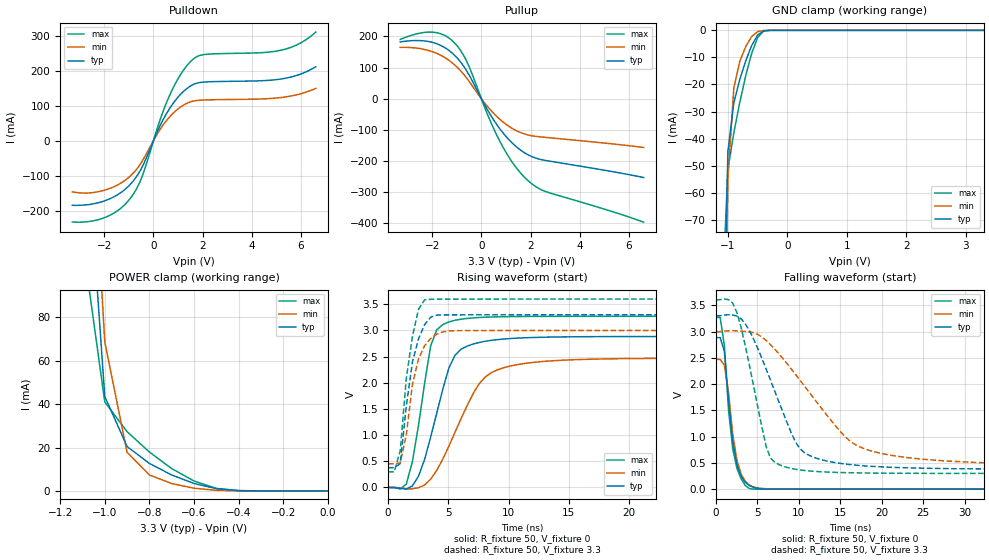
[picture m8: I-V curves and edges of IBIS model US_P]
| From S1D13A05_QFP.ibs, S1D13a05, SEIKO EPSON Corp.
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[Model]   US_P
Model_type I/O
Enable Active-Low
Polarity Non-Inverting
Vinh=2.0
Vinl=0.8
Vref=0
Vmeas=1.65
Rref=500
Cref=100pf
C_comp   5p   4p   6p
[Temperature Range] 25   85   -40
[Voltage Range]   3.3   3.0   3.6
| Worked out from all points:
|   slope of the pulldown table from 0 to 0.495 V, typ, clamps not added: 6.74 ohm
|   slope of the pullup table from 0 to 0.495 V, typ, clamps not added: 7.33 ohm
|   GND clamp passes 1 mA (typ) near -0.45 V on its own axis
|   POWER clamp passes 1 mA (typ) near -0.50 V on its own axis
|   falling waveform, R_fixture 50, V_fixture 0: 20-80 % time 1.22ns typ, 1.25ns min, 1.12ns max; typ from 2.88 V to 0 V
|   falling waveform, R_fixture 50, V_fixture 3.3: 20-80 % time 4.47ns typ, 7.76ns min, 2.62ns max; typ from 3.3 V to 0.379 V
|   rising waveform, R_fixture 50, V_fixture 0: 20-80 % time 2.02ns typ, 3.12ns min, 1.33ns max; typ from 0 V to 2.88 V
|   rising waveform, R_fixture 50, V_fixture 3.3: 20-80 % time 1.14ns typ, 1.12ns min, 971ps max; typ from 0.378 V to 3.3 V
[Pullup]
-3.3V     182mA      164.8mA    189.8mA
-2.6V     186.7mA    161.9mA    208.6mA
-2V       180.8mA    151.1mA    213.4mA
-1.5V     164.5mA    132.5mA    203.4mA
-1.1V     140.1mA    109.3mA    179.6mA
-600mV    89.77mA    66.62mA    120.5mA
300mV     -42.81mA   -29.74mA   -59.99mA
900mV     -111.5mA   -75.9mA    -158.2mA
1.5V      -159.1mA   -105.3mA   -229.4mA
2.1V      -187.1mA   -119.5mA   -275.7mA
2.7V      -199.1mA   -124.6mA   -300mA
6.6V      -252.7mA   -156.2mA   -395.8mA
[Pulldown]
-3.3V     -184.8mA   -146.4mA   -232.6mA
-1.9V     -169.9mA   -139.8mA   -217.7mA
-900mV    -121.6mA   -98.26mA   -161.1mA
-500mV    -80.82mA   -63.36mA   -109.6mA
300mV     47.55mA    35.72mA    66.22mA
700mV     96.96mA    71.67mA    136.6mA
1.1V      132.7mA    96.38mA    189.3mA
1.6V      160.5mA    113.3mA    232.8mA
2.1V      168.2mA    116.8mA    247mA
5.2V      176.9mA    123.8mA    259.4mA
5.9V      188.8mA    132.9mA    276.9mA
6.6V      211.7mA    149.8mA    311.1mA
[GND Clamp]
-3.3V     -5.912A    -5.005A    -7.437A
-1.1V     -148.8mA   -201.2mA   -101.3mA
-1V       -44.75mA   -55.01mA   -51.59mA
-900mV    -26.74mA   -21.22mA   -37.75mA
-800mV    -18.11mA   -11.47mA   -26.61mA
-700mV    -11.25mA   -5.992mA   -16.74mA
-600mV    -5.634mA   -2.285mA   -8.486mA
-500mV    -1.764mA   -477.5uA   -2.648mA
-400mV    -228.7uA   -55.77uA   -273.5uA
-300mV    -14.09uA   -4.898uA   -8.486uA
3.3V      997.8pA    2.959uA    138.9pA
[POWER Clamp]
-3.3V     6.221A     5.265A     7.806A
-1.1V     190.4mA    247mA      115.3mA
-1V       43.51mA    68.6mA     40.98mA
-900mV    20.45mA    17.8mA     27.29mA
-800mV    12.66mA    7.365mA    17.91mA
-700mV    7.343mA    3.399mA    10.28mA
-600mV    3.431mA    1.245mA    4.569mA
-500mV    1.039mA    278.7uA    1.157mA
-400mV    155.6uA    36.37uA    108uA
0V        997.8pA    2.129nA    167.6pA
[Falling Waveform]
R_fixture=50
V_fixture=0
V_fixture_min=0
V_fixture_max=0
0s        2.885V     2.471V     3.271V
505.1ps   2.885V     2.471V     3.27V
1.01ns    2.63V      2.363V     2.739V
1.515ns   1.701V     1.838V     1.505V
2.02ns    902.7mV    1.05V      770.1mV
2.525ns   472.3mV    551.8mV    397.7mV
3.03ns    247.6mV    286.4mV    199.1mV
4.04ns    66.95mV    79.7mV     10.84mV
7.576ns   1.173mV    2.989mV    758.1uV
50ns      4.747uV    28.51uV    6.901uV
[Falling Waveform]
R_fixture=50
V_fixture=3.3
V_fixture_min=3.0
V_fixture_max=3.6
0s        3.3V       3V         3.6V
1.515ns   3.321V     3.015V     3.609V
2.525ns   3.294V     3.014V     3.362V
4.04ns    3.016V     2.995V     2.354V
6.061ns   2.286V     2.831V     810.9mV
7.576ns   1.669V     2.58V      469.6mV
10.61ns   704.3mV    1.978V     357.6mV
15.66ns   477.4mV    989.7mV    314.4mV
18.18ns   440.9mV    756.1mV    307.6mV
50ns      379mV      461.4mV    299mV
[Rising Waveform]
R_fixture=50
V_fixture=0
V_fixture_min=0
V_fixture_max=0
0s        0V         0V         0V
1.515ns   -32.09mV   -25.01mV   64.98mV
2.525ns   215.1mV    -5.291mV   1.185V
3.535ns   963.1mV    158.1mV    2.707V
4.04ns    1.422V     327.8mV    3.012V
5.051ns   2.286V     791.6mV    3.163V
6.061ns   2.642V     1.318V     3.216V
7.576ns   2.772V     1.988V     3.248V
11.11ns   2.858V     2.362V     3.267V
50ns      2.885V     2.471V     3.271V
[Rising Waveform]
R_fixture=50
V_fixture=3.3
V_fixture_min=3.0
V_fixture_max=3.6
0s        378.4mV    453.1mV    299mV
505.1ps   378.6mV    453.2mV    299mV
1.01ns    455.8mV    466.7mV    701.2mV
1.515ns   1.558V     1.007V     2.09V
2.02ns    2.397V     1.966V     2.883V
2.525ns   2.838V     2.458V     3.405V
3.03ns    3.112V     2.709V     3.585V
4.04ns    3.293V     2.93V      3.598V
5.556ns   3.298V     2.996V     3.599V
50ns      3.3V       3V         3.6V
[Ramp]
R_load=50
dV/dt_r   1.731E+0/1.999E-9   1.482E+0/3.104E-9   1.963E+0/1.289E-9
dV/dt_f   1.753E+0/4.451E-9   1.523E+0/7.741E-9   1.981E+0/2.597E-9
